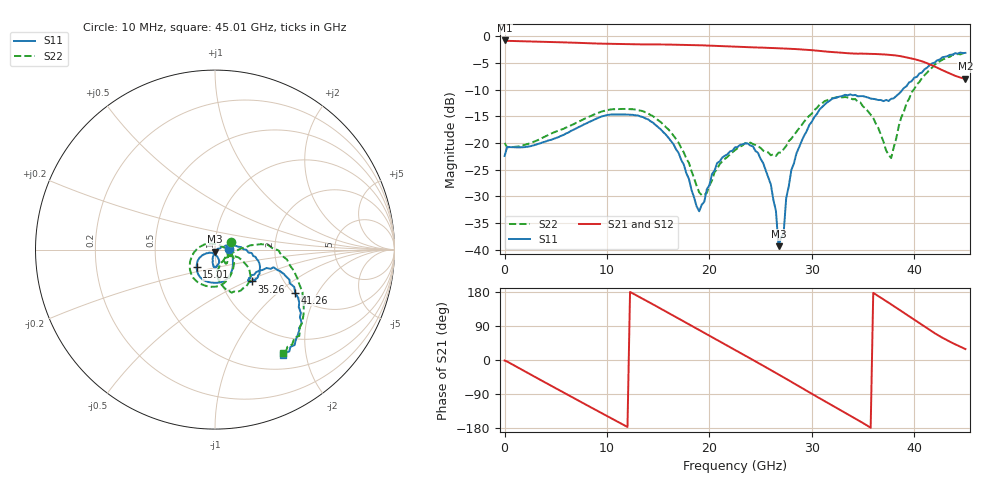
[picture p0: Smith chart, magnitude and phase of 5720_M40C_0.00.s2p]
! Device:  ADRF5720
! Description: 0.5dB LSB GaAs MMIC 6-bit Digital Attenuator
! Frequency:  0.000009 -  40 GHz
! Ports:
!	RF1	= Port 1
!	RF2	= Port 2
! Vdd:  3.3 Volt
! Vss:  -3.3 Volt
! Control:  0/3.3 Volt
! State:  0.00 dB attenuation
! Data:  The device was measured using G-S-G Probes on a matrix board.
!  Data was collected using an calibrated 4 port network analyzer.
!  The reference plane for this measurement is at the launchers.
! Note:  Analog Devices supplies this data as a sample of measured data
!  for this product.  Your particular data for this product may vary.
!  Data was taken at -40 degrees C.
!  Analog Devices reserves the right to change this data at anytime.
# GHZ S DB R 45.0
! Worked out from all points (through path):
!   181 points, 10 MHz to 45.01 GHz, reference 45 ohm
!   highest |S21| = -0.80 dB at 10 MHz (marker M1); lowest = -8.0 dB at 45.01 GHz (marker M2)
!   group delay of S21, straight-line fit = 42.6 ps
!   lowest |S11| = -39.3 dB at 26.76 GHz (marker M3), VSWR 1.02, Z = 45 - j0.972 ohm
!   |S11| at or under -10 dB: start of sweep to 38.88 GHz
!   |S22| runs from -29.8 to -3.2 dB; largest |S21 - S12| = 0.0033
!   S11 on the Smith chart (normalised r, x): 10 MHz: 1.16, +0.01; 15.01 GHz: 0.80, -0.16; 35.26 GHz: 1.39, -0.53; 41.26 GHz: 2.04, -1.32; 45.01 GHz: 0.70, -1.61
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0.01  -22.44 3.3  -0.80 -1.4  -0.82 -1.4  -20.00 24.5
4.26  -19.54 -22.0  -1.08 -63.6  -1.10 -63.6  -18.49 -27.3
7.76  -16.52 -50.7  -1.28 -115.0  -1.30 -115.1  -15.52 -58.7
11.51  -14.67 -92.8  -1.48 -169.5  -1.50 -169.6  -13.63 -101.9
15.01  -17.07 -136.8  -1.55 139.2  -1.57 139.2  -15.74 -149.1
15.26  -17.47 -139.6  -1.55 135.5  -1.57 135.4  -16.10 -152.9
17.01  -21.90 -155.6  -1.60 109.3  -1.62 109.3  -19.98 177.7
19.01  -32.80 -116.8  -1.70 79.2  -1.72 79.1  -29.24 106.8
20.76  -23.78 -68.8  -1.83 52.8  -1.85 52.7  -24.90 2.6
22.76  -20.76 -84.4  -1.99 22.7  -2.01 22.6  -20.99 -36.5
25.26  -23.75 -100.2  -2.15 -15.1  -2.17 -15.2  -21.43 -52.4
26.51  -32.76 -96.6  -2.24 -34.3  -2.26 -34.4  -22.44 -38.4
26.76  -39.33 -88.1  -2.26 -38.1  -2.28 -38.3  -21.80 -32.3
27.26  -36.92 17.8  -2.29 -45.9  -2.31 -46.0  -21.16 -24.2
27.51  -30.32 13.8  -2.31 -49.7  -2.33 -49.9  -20.57 -23.1
28.01  -25.07 19.5  -2.36 -57.6  -2.38 -57.7  -19.20 -20.2
30.26  -15.14 -0.4  -2.66 -93.0  -2.69 -93.2  -13.83 -27.5
35.26  -11.36 -41.1  -3.27 -170.4  -3.30 -170.6  -13.55 -77.8
37.76  -11.73 -32.6  -3.52 146.9  -3.55 146.7  -22.83 -35.9
39.26  -9.36 -16.8  -3.98 120.0  -4.00 119.8  -12.52 6.7
41.26  -5.91 -28.2  -5.07 83.7  -5.09 83.6  -6.85 -15.0
45.01  -3.13 -57.1  -7.96 28.8  -7.99 28.7  -3.24 -56.7
